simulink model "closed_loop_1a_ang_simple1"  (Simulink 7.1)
settings: Solver=FixedStepDiscrete  StartTime=0.0  StopTime=Tend  FixedStep=Ts  MaxStep=Ts  MinStep=Ts/10  RelTol=1e-4
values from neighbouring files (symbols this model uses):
  Kt = 0.06    [lame_dat.m]
  Ts = 100e-6    (= 0.0001)    [lame_main.m]
undefined symbols (not defined in the file or in its folder): A
libraries: powerlib_extras x1, cstblocks x1

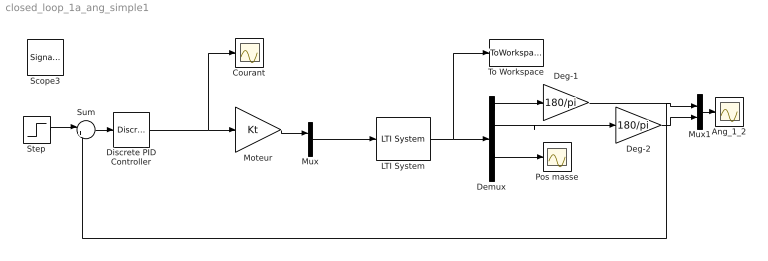
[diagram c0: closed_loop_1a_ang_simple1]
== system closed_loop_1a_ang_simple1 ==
  Ang_1_2 : Scope
  Courant : Scope
  Deg-1 : Gain  Gain=180/pi  ParameterDataType=fixdt(1, 16)  ParameterScaling=2^0  OutDataType=fixdt(1, 16)  OutScaling=2^0
  Deg-2 : Gain  Gain=180/pi  ParameterDataType=fixdt(1, 16)  ParameterScaling=2^0  OutDataType=fixdt(1, 16)  OutScaling=2^0
  Demux : Demux  Outputs=5
  Discrete PID Controller : powerlib_extras/Discrete  Control Blocks/Discrete PID Controller  DialogController=POWERSYS.PowerSysDialog  SystemSampleTime=-1  Kp=20  Ki=50  Kd=0.002  TcD=Ts  Par_Limits="[1    -1]"  Init=0  Ts=Ts
  LTI System : cstblocks/LTI System  SystemSampleTime=-1  sys=sysd  IC=[]
  Moteur : Gain  Gain=Kt  ParameterDataType=sfix(16)  ParameterScaling=2^0  OutDataType=sfix(16)  OutScaling=2^0
  Mux : Mux  Inputs=2
  Mux1 : Mux  Inputs=2
  Pos masse : Scope
  Step : Step  Time=0  After=A  SampleTime=0
  Sum : Sum  Inputs=|+-  OutDataType=sfix(16)  OutScaling=2^0
  To Workspace : ToWorkspace  VariableName=y_sim_out  SampleTime=-1  SaveFormat=Structure With Time
  Scope3 : SignalViewerScope  IOType=viewer  RefreshTime=0.035000
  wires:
  LTI System/1 -> Demux/1, To Workspace/1
  Demux/1 -> Deg-1/1
  Moteur/1 -> Mux/1
  Mux/1 -> LTI System/1
  Step/1 -> Sum/1
  Sum/1 -> Discrete PID Controller/1
  Discrete PID Controller/1 -> Moteur/1, Courant/1
  Demux/4 -> Pos masse/1
  Demux/2 -> Deg-2/1
  Mux1/1 -> Ang_1_2/1
  Deg-1/1 -> Mux1/1, Sum/2
  Deg-2/1 -> Mux1/2
